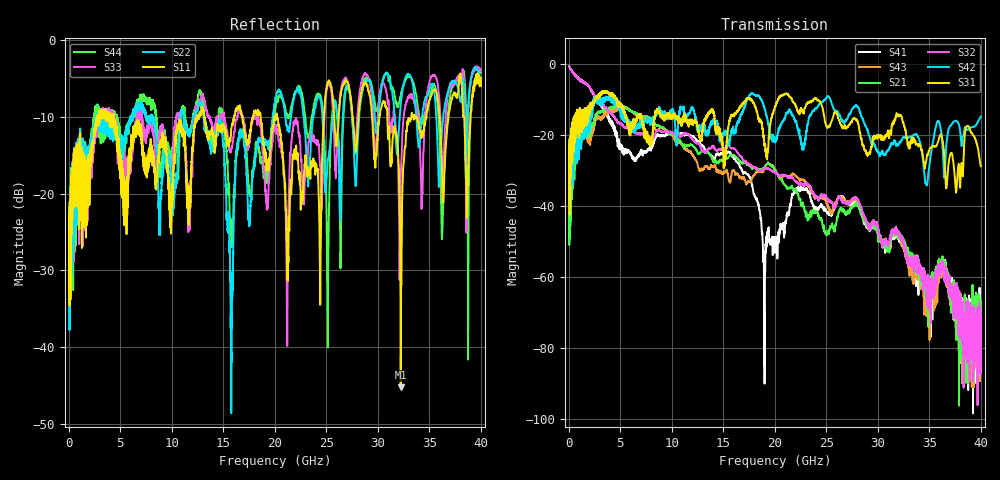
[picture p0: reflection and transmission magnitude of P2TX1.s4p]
!Agilent Technologies,N5245A,MY49151084,A.09.20.08
!Agilent N5245A: A.09.20.08
!Date: Thursday, March 01, 2012 10:27:21
!Correction: S11(Full 4 Port(1,2,3,4))
!S12(Full 4 Port(1,2,3,4))
!S13(Full 4 Port(1,2,3,4))
!S14(Full 4 Port(1,2,3,4))
!S21(Full 4 Port(1,2,3,4))
!S22(Full 4 Port(1,2,3,4))
!S23(Full 4 Port(1,2,3,4))
!S24(Full 4 Port(1,2,3,4))
!S31(Full 4 Port(1,2,3,4))
!S32(Full 4 Port(1,2,3,4))
!S33(Full 4 Port(1,2,3,4))
!S34(Full 4 Port(1,2,3,4))
!S41(Full 4 Port(1,2,3,4))
!S42(Full 4 Port(1,2,3,4))
!S43(Full 4 Port(1,2,3,4))
!S44(Full 4 Port(1,2,3,4))
!S4P File: Measurements: <S11,S12,S13,S14>,
!<S21,S22,S23,S24>,
!<S31,S32,S33,S34>,
!<S41,S42,S43,S44>:
# Hz S  dB  R 50
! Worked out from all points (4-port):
!   3996 points, 50 MHz to 40 GHz, reference 50 ohm
!   strongest paths, dB at 50 MHz, 10.04 GHz, 20.03 GHz, 30.02 GHz, 40 GHz:
!     S31: -27.3, -14.5, -11.9, -20.5, -28.9
!     S42: -26.9, -13.3, -22.2, -25.1, -14.8
!     S32: -0.8, -19.5, -30.7, -46.3, -75.6
!     S21: -49.6, -19.6, -30.0, -48.4, -69.3
!     S43: -46.4, -19.7, -29.9, -48.3, -73.8
!     S41: -0.7, -19.9, -49.1, -46.9, -68.2
!   lowest |S11| = -45.2 dB at 32.22 GHz (marker M1), VSWR 1.01, Z = 49.8 - j0.517 ohm
!   |S11| at or under -10 dB: 4.38 GHz to 12.49 GHz (8.105 GHz wide, 96.1 % of centre); 13.17 GHz to 16.05 GHz (2.88 GHz wide, 19.7 % of centre); 20.21 GHz to 24.77 GHz (4.563 GHz wide, 20.3 % of centre)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
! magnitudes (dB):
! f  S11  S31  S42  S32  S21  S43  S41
! 50 MHz  -24.6  -27.3  -26.9  -0.8  -49.6  -46.4  -0.7
! 4.89 GHz  -15.2  -11.3  -12.3  -16.7  -11.8  -12.3  -23.9
! 15.78 GHz  -11.5  -14.6  -19.0  -23.8  -25.7  -31.8  -25.7
! 19 GHz  -14.4  -22.6  -12.4  -29.6  -29.3  -29.6  -75.7
! 22.18 GHz  -15.6  -13.0  -17.5  -33.5  -36.4  -32.0  -35.3
! 32.22 GHz  -45.2  -14.5  -22.2  -49.2  -48.2  -49.7  -50.4
! 40 GHz  -6.0  -28.9  -14.8  -75.6  -69.3  -73.8  -68.2
